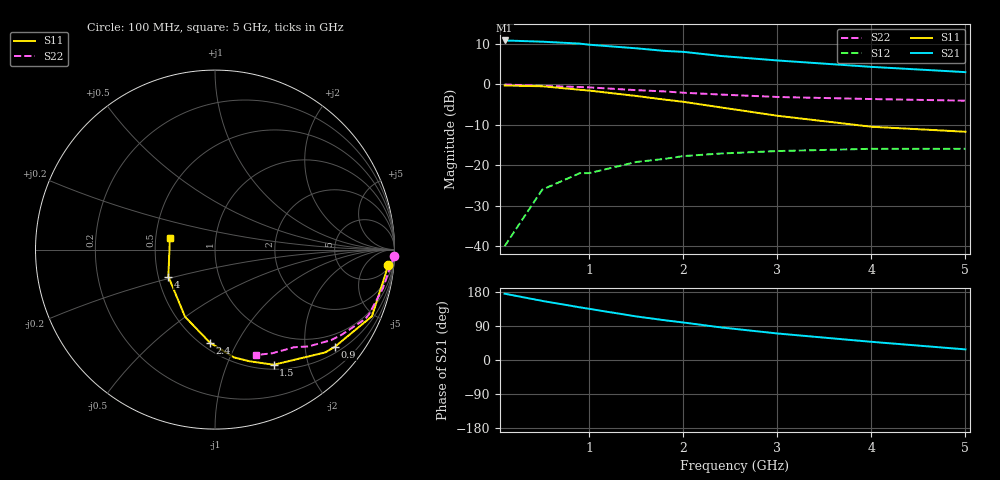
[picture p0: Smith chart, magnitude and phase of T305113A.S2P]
!AT-30511
!S and NOISE PARAMETERS at Vce=2.7V  Ic=1mA.  LAST UPDATED 06-23-94
# ghz s ma r 50
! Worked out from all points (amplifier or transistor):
!   11 points, 100 MHz to 5 GHz, reference 50 ohm
!   highest |S21| = 10.9 dB at 100 MHz (marker M1)
!   |S21| within 3 dB of that: start of sweep to 2.071 GHz
!   unconditionally stable (mu >= 1): 3.674 GHz to end of sweep
!   at 500 MHz: K = 0.17, MSG = 18.3 dB, |S12| = -26.0 dB
!   at 1.8 GHz: K = 0.56, MSG = 13.4 dB, |S12| = -18.4 dB
!   at 5 GHz: K = 1.24, MAG = 6.5 dB, |S12| = -15.9 dB
!   lowest NFmin = 0.30 dB at 500 MHz
!   S11 on the Smith chart (normalised r, x): 100 MHz: 7, -20; 900 MHz: 0.65, -2.69; 1.5 GHz: 0.56, -1.48; 2.4 GHz: 0.55, -0.78; 4 GHz: 0.57, -0.19; 5 GHz: 0.59, +0.09
0.1  0.97 -5.0  3.5 175.0  0.01 86.0  0.999 -2.0
0.5  0.95 -23.0  3.38 156.0  0.05 74.0  0.96 -13.0
0.9  0.86 -39.0  3.2 139.0  0.08 63.0  0.93 -23.0
1  0.84 -43.0  3.1 135.0  0.08 60.0  0.92 -25.0
1.5  0.72 -63.0  2.8 115.0  0.11 49.0  0.85 -34.0
1.8  0.65 -73.0  2.6 105.0  0.12 43.0  0.82 -38.0
2  0.61 -80.0  2.53 99.0  0.13 40.0  0.79 -41.0
2.4  0.52 -93.0  2.25 86.0  0.14 35.0  0.75 -46.0
3  0.41 -114.0  1.98 70.0  0.15 30.0  0.7 -51.0
4  0.3 -150.0  1.65 48.0  0.16 23.0  0.66 -61.0
5  0.26 165.0  1.42 28.0  0.16 22.0  0.63 -69.0
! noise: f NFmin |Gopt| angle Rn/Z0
0.5  0.3  0.96  10  1.49
0.9  0.4  0.92  19  1.33
1.8  0.9  0.83  43  0.98
2.4  1.3  0.76  60  0.74
